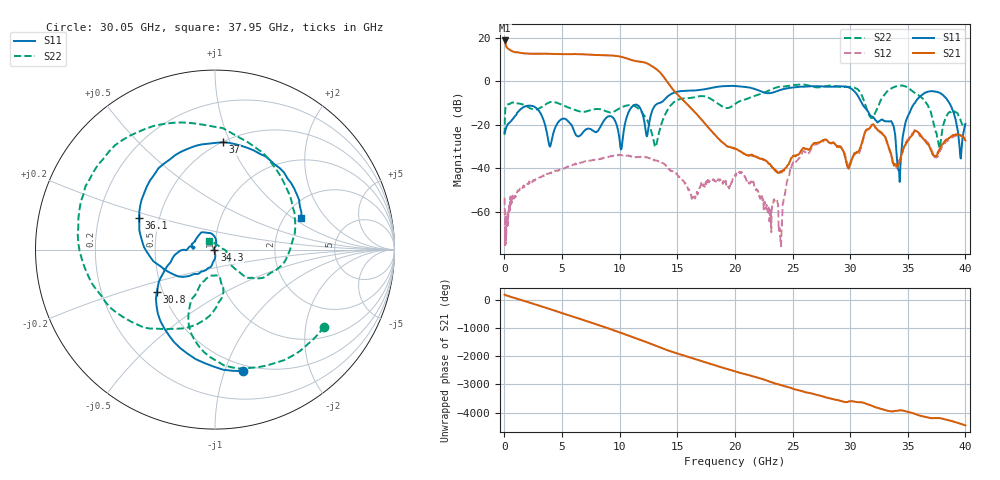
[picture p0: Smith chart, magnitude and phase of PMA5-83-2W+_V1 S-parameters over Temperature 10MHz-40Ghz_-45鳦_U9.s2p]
!Mini-Circuits Laboratory
!S-Parameters
!Model: US-AMP-1
!Run / Lot / Date Code: N/A / N/A / N/A
!Fixture: N/A, Pressing Arm: N/A
!Network Analyzer: NFA N8975A;  Serial number: 74408
!Date: 11/29/2023 at 10:17:49 AM
!No.: Unit# 2 (U9)
!Tested with: -45°C
! 2 port cal with Bias Tee PE1622 in line. No normalization applied. Bias cond 2: Vdd= 12V, Idd= 400mA, Vg2= 5V, starting point for Vg1= -2V
# Hz  S  dB  R  50
!Frequency  S11 dB  S11 Deg  S21 dB  S21 Deg  S12 dB  S12 Deg  S22 dB  S22 Deg
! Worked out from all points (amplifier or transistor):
!   826 points, 10 MHz to 40 GHz, reference 50 ohm
!   highest |S21| = 18.9 dB at 20 MHz (marker M1)
!   |S21| within 3 dB of that: start of sweep to 175 MHz
!   unconditionally stable (mu >= 1): start of sweep to end of sweep
!   at 5.6 GHz: K = 10.14, MAG = 12.9 dB, |S12| = -39.4 dB
!   at 19.4 GHz: K = 1502.86, MAG = -25.5 dB, |S12| = -48.5 dB
!   at 40 GHz: K = 243.71, MAG = -27.1 dB, |S12| = -26.8 dB
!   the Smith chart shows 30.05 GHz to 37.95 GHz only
!   S11 on the Smith chart (normalised r, x): 30.05 GHz: 0.44, -1.15; 30.8 GHz: 0.46, -0.26; 34.3 GHz: 0.99, -0.01; 36.1 GHz: 0.38, +0.17; 37 GHz: 0.50, +0.94; 37.95 GHz: 2.47, +1.16
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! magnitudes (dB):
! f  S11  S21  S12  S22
! 10 MHz  -23.5  18.9  -53.6  -24.6
! 20 MHz  -23.2  18.9  -58.3  -20.3
! 2.15 GHz  -11.1  12.8  -46.0  -12.1
! 3.95 GHz  -30.0  12.7  -42.0  -9.5
! 6.7 GHz  -24.2  12.6  -37.2  -14.0
! 10.1 GHz  -31.3  11.4  -33.9  -12.0
! 13.35 GHz  -10.0  5.0  -36.7  -25.0
! 16.35 GHz  -4.2  -13.2  -52.3  -7.4
! 20.05 GHz  -2.1  -31.1  -43.7  -10.2
! 23.95 GHz  -3.9  -41.4  -74.1  -2.4
! 24.95 GHz  -2.8  -35.0  -38.5  -1.8
! 26.7 GHz  -2.2  -29.4  -30.3  -2.2
! 30.05 GHz  -3.2  -37.5  -36.6  -2.6
! 30.8 GHz  -7.9  -31.6  -32.7  -4.4
! 31.85 GHz  -16.0  -20.2  -20.4  -16.7
! 33.35 GHz  -18.5  -30.3  -30.9  -4.0
! 34.3 GHz  -46.3  -37.0  -36.0  -1.9
! 36.1 GHz  -6.8  -24.8  -24.5  -6.9
! 37 GHz  -4.4  -31.6  -30.8  -14.1
! 37.95 GHz  -5.8  -29.2  -30.4  -24.2
! 39.55 GHz  -34.3  -24.6  -24.9  -17.2
! 40 GHz  -19.6  -27.1  -26.8  -20.4
